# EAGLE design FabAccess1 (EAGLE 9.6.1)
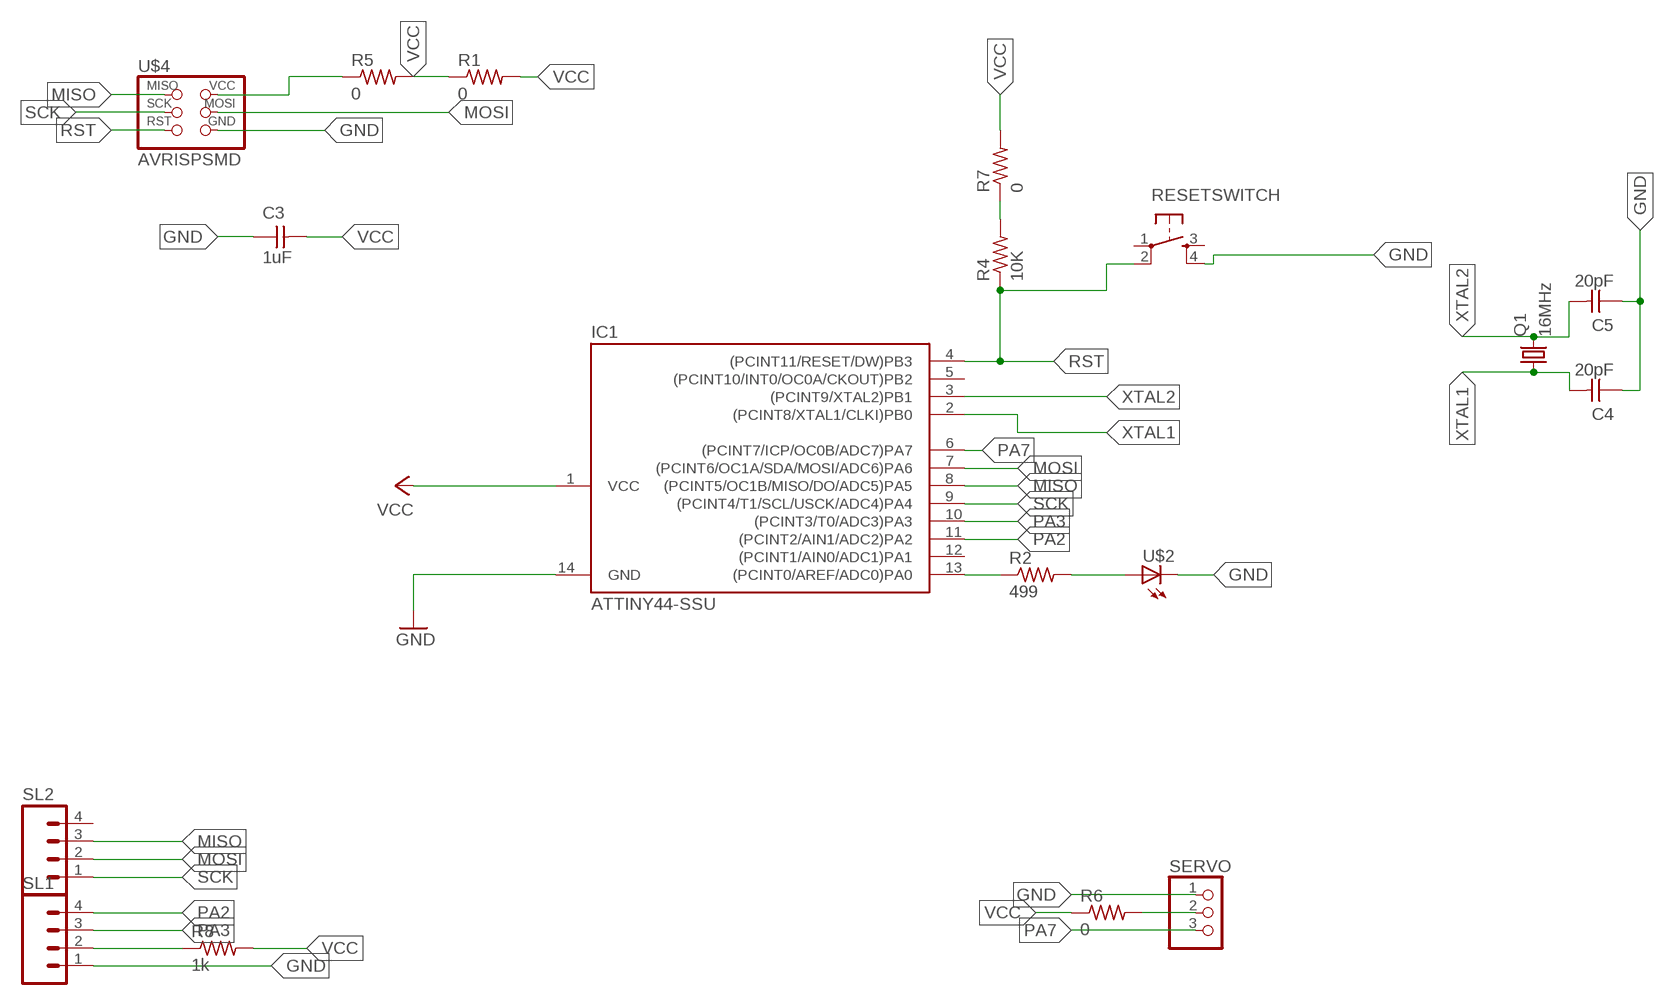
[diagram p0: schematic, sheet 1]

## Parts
C3  1uF  UNPOLARIZED_CAPACITOR1206  [1206]
C4  20pF  UNPOLARIZED_CAPACITOR1206  [1206]
C5  20pF  UNPOLARIZED_CAPACITOR1206  [1206]
IC1  ATTINY44-SSU  [SOIC14]
Q1  16MHz  CSM-7X-DU  [CSM-7X-DU]
R1  0  RES-US1206  [R1206]
R2  499  RES-US1206  [R1206]
R4  10K  RESISTOR1206  [1206]
R5  0  RES-US1206  [R1206]
R6  0  RES-US1206  [R1206]
R7  0  RESISTOR1206  [1206]
R8  1k  RES-US1206  [R1206]
RESETSWITCH  6MM_SWITCH6MM_SWITCH  [6MM_SWITCH]
SERVO  PINHD-1X3  [1X03]
SL1  M04  [04P]
SL2  M04  [04P]
U$2  LED1206  [1206]
U$4  AVRISPSMD  [2X03SMD]

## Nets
GND: C3.1 C4.1 C5.1 IC1.14(GND) RESETSWITCH.4(S1) SERVO.1 SL1.1 U$2.2(C) U$4.6(GND)
MISO: IC1.8((PCINT5/OC1B/MISO/DO/ADC5)PA5) SL2.3 U$4.1(MISO)
MOSI: IC1.7((PCINT6/OC1A/SDA/MOSI/ADC6)PA6) SL2.2 U$4.4(MOSI)
N$1: IC1.13((PCINT0/AREF/ADC0)PA0) R2.1
N$2: R2.2 U$2.1(A)
N$3: R8.1 SL1.2
N$5: R4.2 R7.1
PA2: IC1.11((PCINT2/AIN1/ADC2)PA2) SL1.4
PA3: IC1.10((PCINT3/T0/ADC3)PA3) SL1.3
PA7: IC1.6((PCINT7/ICP/OC0B/ADC7)PA7) SERVO.3
RST: IC1.4((PCINT11/RESET/DW)PB3) R4.1 RESETSWITCH.2(P1) U$4.5(RST)
SCK: IC1.9((PCINT4/T1/SCL/USCK/ADC4)PA4) SL2.1 U$4.3(SCK)
VCC: C3.2 IC1.1(VCC) R1.1 R1.2 R5.1 R5.2 R6.1 R6.2 R7.2 R8.2 SERVO.2 U$4.2(VCC)
XTAL1: C4.2 IC1.2((PCINT8/XTAL1/CLKI)PB0) Q1.1
XTAL2: C5.2 IC1.3((PCINT9/XTAL2)PB1) Q1.2
Unconnected: IC1.5((PCINT10/INT0/OC0A/CKOUT)PB2) IC1.12((PCINT1/AIN0/ADC1)PA1) RESETSWITCH.1(P) RESETSWITCH.3(S) SL2.4

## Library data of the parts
C3-C5 = FAB_Hello:UNPOLARIZED_CAPACITOR: unpolarized_capacitor
IC1 = FAB_Hello:ATTINY44
Q1 = FAB_Hello:CSM-7X-DU: SMD CRYSTAL; OC_FARNELL: unknown; OC_NEWARK: unknown
R1 R2 R5 R6 R8 = fab:RES-US: Resistor (US Symbol)
R4 R7 = FAB_Hello:RESISTOR
RESETSWITCH = FAB_Hello:6MM_SWITCH: OMRON SWITCH
SERVO = pinhead:PINHD-1X3: PIN HEADER
SL1 SL2 = con-amp-quick:M04: AMP QUICK CONNECTOR; OC_FARNELL: unknown; OC_NEWARK: unknown
U$2 = FAB_Hello:LED
U$4 = FAB_Hello:AVRISP

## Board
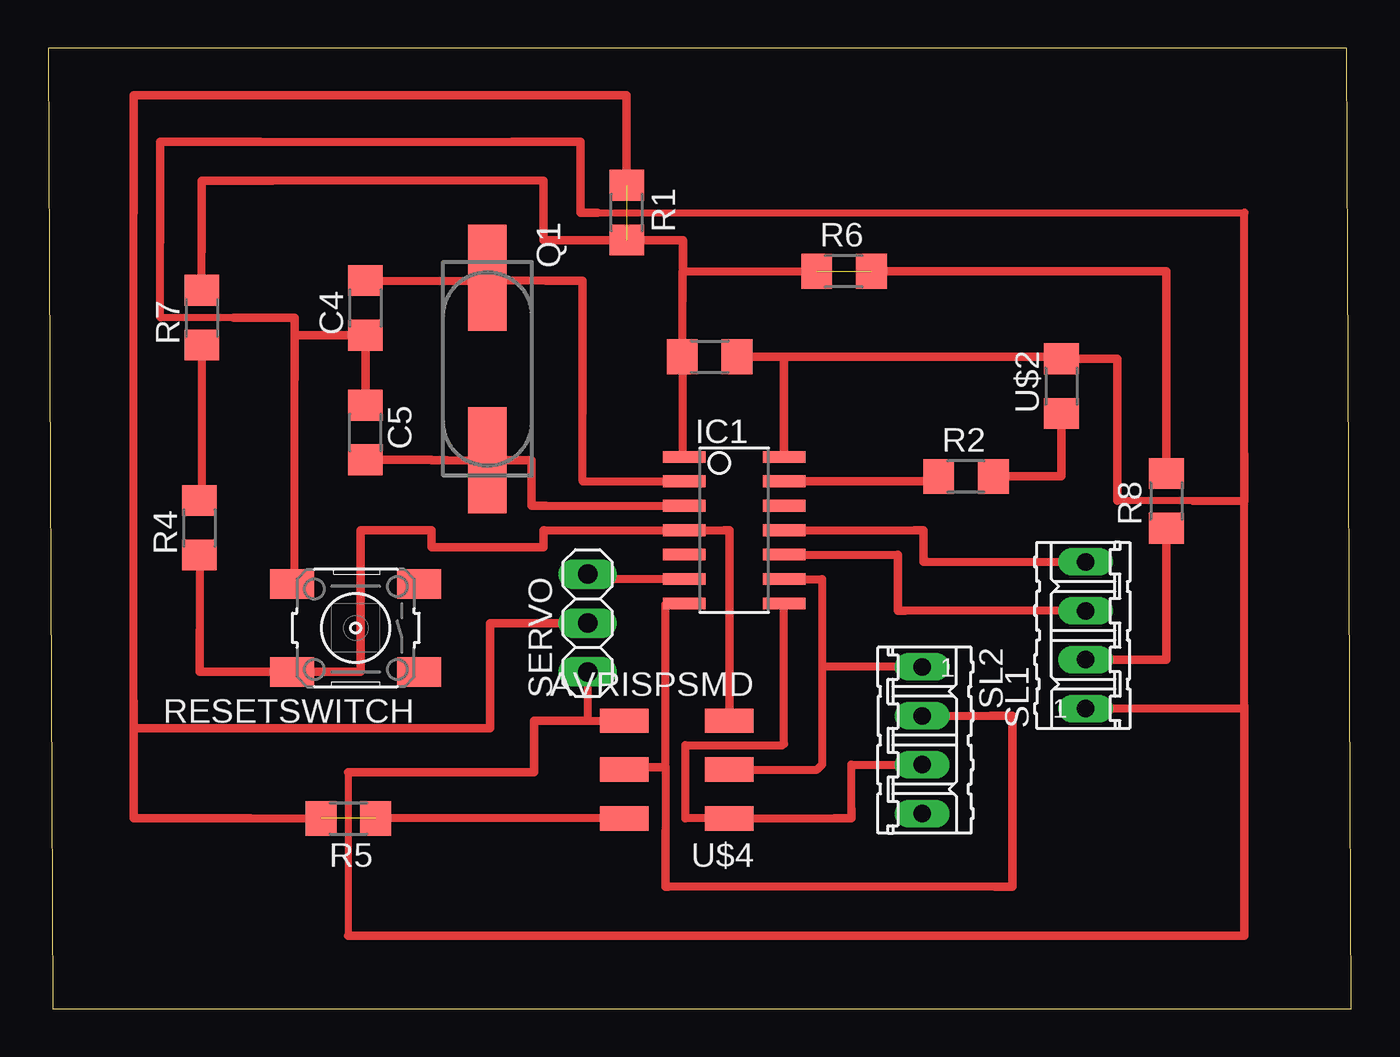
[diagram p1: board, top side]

Size 67.8 x 49.96 mm. Coordinates in mm from the lower left corner, seen from the top.
Outline: 0.25,0 67.8,0 67.54,49.96 0,49.96 0.25,0
Copper layers (1*16): Top 0.035mm / dielectric 1.5mm / Bottom 0.035mm
Design rules "default *": minimum track width 6mil, minimum drill 0.35mm, track to track 17mil, track to pad 17mil, pad to pad 17mil, via to via 17mil, smd to smd 17mil, copper to edge 40mil, drill to drill 6mil, minimum pad ring 10mil, minimum via ring 8mil, stop-mask expansion 4mil, vias tented up to drill 0mil, thermal gap 17mil

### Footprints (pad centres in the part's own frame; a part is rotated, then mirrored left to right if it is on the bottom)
1206 = smd 1.6 x 1.803: 1 -1.422,0; 2 1.422,0
SOIC14 = smd 0.61 x 2.21: 1 -3.81,-2.603; 2 -2.54,-2.603; 3 -1.27,-2.603; 4 0,-2.603; 5 1.27,-2.603; 6 2.54,-2.603; 7 3.81,-2.603; 8 3.81,2.603; 9 2.54,2.603; 10 1.27,2.603; 11 0,2.603; 12 -1.27,2.603; 13 -2.54,2.603; 14 -3.81,2.603
CSM-7X-DU = smd 5.5 x 2: 1 -4.75,0; 2 4.75,0
R1206 = smd 1.6 x 1.803: 1 -1.422,0; 2 1.422,0
6MM_SWITCH = smd 2.286 x 1.524: 1 -3.302,2.286; 2 3.302,2.286; 3 -3.302,-2.286; 4 3.302,-2.286
1X03 = drill 1.016 long: 1 -2.54,0; 2 0,0; 3 2.54,0
04P = drill 0.914 long: 1 -3.81,0; 2 -1.27,0; 3 1.27,0; 4 3.81,0
2X03SMD = smd 2.54 x 1.27: 1 -2.54,2.54; 2 2.92,2.54; 3 -2.54,0; 4 2.92,0; 5 -2.54,-2.54; 6 2.92,-2.54

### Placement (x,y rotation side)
C3  34.42,33.91 180 top
C4  16.51,36.45 90 top
C5  16.51,29.97 270 top
IC1  35.69,24.89 270 top
Q1  22.86,33.27 270 top
R1  30.1,41.4 270 top
R2  47.75,27.69 0 top
R4  7.87,25.02 90 top
R5  15.62,9.91 180 top
R6  41.4,38.35 0 top
R7  8,35.94 90 top
R8  58.17,26.42 90 top
RESETSWITCH  16,19.81 180 top
SERVO  28.07,20.07 90 top
SL1  53.98,19.43 90 top
SL2  45.47,13.97 270 top
U$2  52.71,32.38 90 top
U$4  32.89,12.45 180 top

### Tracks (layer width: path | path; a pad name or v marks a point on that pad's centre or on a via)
GND
  Top 0.356: 59.56,26.42 55.63,26.42 | 28.57,41.4 62.23,41.4 | 9.65,35.94 5.84,35.94 | 15.62,12.32 15.62,3.81
  Top 0.406: RESETSWITCH.4 12.83,22.23 12.83,32.77 | U$4.6 28.07,14.99 SERVO.1 | 59.56,26.42 62.23,26.42 62.23,15.75 62.1,15.62 SL1.1 | 62.23,28.83 62.23,41.4 | 11.05,45.09 24.13,45.09 | 5.84,35.94 5.84,39.88
  Top 0.432: 15.62,3.81 62.23,3.81 62.23,15.75 | C3.1 38.29,33.91 | 38.29,33.91 IC1.14 | 38.29,33.91 52.71,33.91 U$2.2 55.63,33.81 55.63,26.42 | 28.07,14.99 25.27,14.99 25.27,12.32 15.62,12.32 | 62.23,26.42 62.23,28.83 | C5.1 C4.1 12.83,35.03 | 12.83,32.77 12.83,35.03 | 12.83,35.03 12.83,35.94 9.65,35.94 | 5.84,39.88 5.84,45.09 11.05,45.09 | 28.57,41.4 27.69,41.4 27.69,45.09 24.13,45.09
MISO
  Top 0.406: 41.27,9.91 40.89,9.91 U$4.1 33.15,9.91 33.15,13.72 38.23,13.72 38.29,13.78 IC1.8 | 41.78,10.41 41.78,12.7 SL2.3
  Top 0.432: 40.89,9.91 41.78,9.91 41.78,10.41
MOSI
  Top 0.406: IC1.7 32.13,21.08 32.13,12.57 32.13,9.27 | SL2.2 49.02,15.24 | 49.28,6.35 32.26,6.35 32.13,6.48
  Top 0.432: U$4.4 30.1,12.57 32.13,12.57 | 32.13,9.27 32.13,6.35 32.26,6.35 | 49.02,15.24 50.16,15.24 50.16,6.35 49.28,6.35
N$1
  Top 0.432: IC1.13 46.33,27.43 R2.1
N$2
  Top 0.432: U$2.1 52.71,27.69 R2.2
N$3
  Top 0.432: SL1.2 58.17,18.16 R8.1
N$5
  Top 0.406: R7.1 8,26.57 R4.2
PA2
  Top 0.406: IC1.11 45.09,24.89 | 45.72,23.24 SL1.4
  Top 0.432: 45.72,23.24 45.53,23.24 45.53,24.89 45.09,24.89
PA3
  Top 0.406: SL1.3 44.58,20.7 | IC1.10 44.2,23.62
  Top 0.432: 44.58,20.7 44.2,20.7 44.2,23.62
PA7
  Top 0.406: IC1.6 28.32,22.35 SERVO.3
RST
  Top 0.406: R4.1 7.87,19.69 | 25.78,24.89 IC1.4 35.18,24.89
  Top 0.432: 25.78,24.89 25.78,24 19.94,24 19.94,24.89 16.26,24.89 16.26,17.53 RESETSWITCH.2 7.87,17.53 7.87,19.69 | 35.18,24.89 35.43,24.89 U$4.5
SCK
  Top 0.406: U$4.3 40.01,12.45 40.26,12.7 40.26,17.78 | IC1.9 40.26,22.35 40.26,17.78 | SL2.1 40.26,17.78
VCC  (3 unrouted)
  Top 0.406: IC1.1 32.99,28.79 C3.2 32.99,36.83 | U$4.2 R5.1 | 30.2,39.88 R1.2 30,39.88 | 33.02,38.35 R6.1 | 10.29,9.91 10.54,9.91 R5.2 | 4.45,15.75 4.45,16 4.45,41.4 | R7.2 8,39.4 | 25.78,43.05 11.66,43.05
  Top 0.432: 32.99,36.83 32.99,38.33 33.02,38.35 33.02,39.98 R1.2 25.78,39.98 25.78,43.05 | R8.2 58.17,38.35 R6.2 | SERVO.2 22.99,20.07 22.99,14.6 4.45,14.6 | 4.45,16 4.45,14.6 | 4.45,14.6 4.45,9.91 10.54,9.91 | 8,39.4 8,43.05 11.66,43.05 | 4.45,41.4 4.45,47.5 30.1,47.5 R1.1
XTAL1
  Top 0.406: IC1.2 27.81,27.43 27.81,30.99 | 22.71,37.87 Q1.1 | 25.88,37.87 22.71,37.87 | C4.2 22.71,37.87
  Top 0.432: 27.81,30.99 27.81,37.87 25.88,37.87
XTAL2
  Top 0.406: 25.91,26.16 IC1.3 | 20.75,28.52 Q1.2 23.55,28.52
  Top 0.432: 20.75,28.52 19.94,28.52 19.94,28.55 C5.2 | 25.91,26.16 25.15,26.16 25.15,28.52 Q1.2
